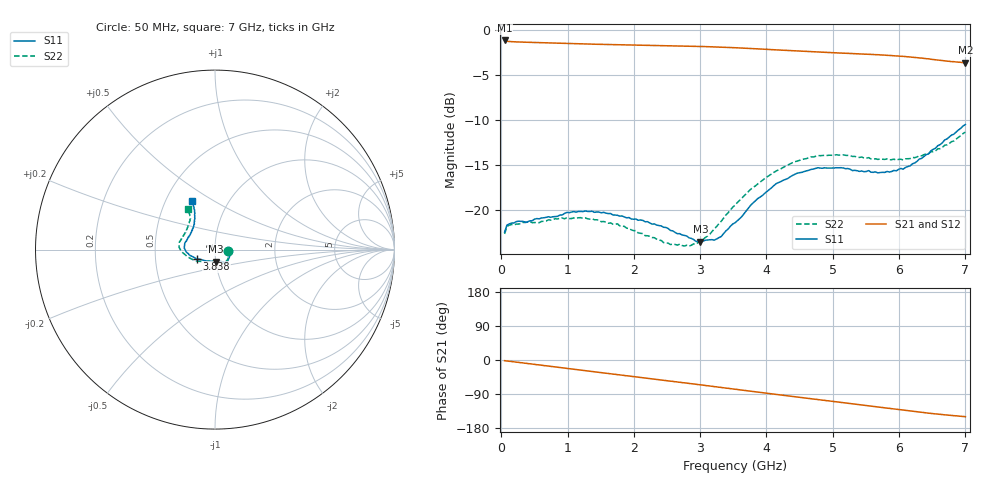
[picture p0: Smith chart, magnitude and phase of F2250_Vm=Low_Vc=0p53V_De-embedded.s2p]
! Integrated Device Technology
! Corporate Headquarters
! 6024 Silver Creek Valley Road
! San Jose, CA 95138  USA
! Phone:  1-408-284-8200
! Toll Free:  1-800-223-1366
! Webpage:  http://www.idt.com/
! Timing and RF Division
! 515 Groton Road, Suite 102
! Westford, MA 01886-6024
! Device:  F2250
! Description: Voltage Variable RF Attenuator
! Frequency:  50.0 -  6000.00 MHz
! Package:  3x3 mm Thin QFN Plastic Package: 16 pin
! Ports:  2 RF, 3 DC
!  Pin  1  = GND
!  Pin  2  = NC
!  Pin  3  = RF1  = Port 1
!  Pin  4  = NC
!  Pin  5  = GND
!  Pin  6  = GND
!  Pin  7  = GND
!  Pin  8  = GND
!  Pin  9  = NC
!  Pin 10  = RF2  = Port 2
!  Pin 11  = NC
!  Pin 12  = GND
!  Pin 13  = GND
!  Pin 14  = VCNTRL
!  Pin 15  = VDD
!  Pin 16  = VMODE
! Vcntrl:  0.530 Volts
! Vmode:  +0.000 Volts
! Vdd:  +3.30  Volts
! Current:  1.130 mA
! Data:  The device was measured on a the F2250 evaluation board which has
!  individual transmission lines to the RF pins.  Data was collected
!  using a calibrated network analyzer.  The evaluation board was
!  de-embedded using a TRL calibration technique.
!  The reference plane is the edge of the package pin.
! Misc:  SN 10
!  Action Tracker AT0258
! Date Measured:  2014-11-26
! Date:  2015-10-15  MJV
! Note:
!  Integrated Device Technology supplies this data as a sample of measured
!  data at the package pin for this product.  Your particular data for this
!  product may vary.
!  Data was taken at 25 degrees C.
!  Integrated Device Technology reserves the right to change this data at anytime.
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# GHz S dB R 50
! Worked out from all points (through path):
!   201 points, 50 MHz to 7 GHz, reference 50 ohm
!   highest |S21| = -1.12 dB at 50 MHz (marker M1); lowest = -3.6 dB at 7 GHz (marker M2)
!   group delay of S21, straight-line fit = 60.1 ps
!   lowest |S11| = -23.5 dB at 3.004 GHz (marker M3), VSWR 1.14, Z = 50 - j6.68 ohm
!   |S11| at or under -10 dB: start of sweep to end of sweep
!   |S22| runs from -24.0 to -11.3 dB; largest |S21 - S12| = 0.00041
!   S11 on the Smith chart (normalised r, x): 50 MHz: 1.16, -0.02; 3.838 GHz: 0.81, -0.08; 7 GHz: 0.68, +0.40
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0.05  -22.45 -7.3  -1.12 -1.8  -1.12 -1.8  -22.66 -8.3
0.08475  -21.68 -7.4  -1.20 -2.5  -1.20 -2.5  -21.83 -7.7
0.15425  -21.45 -9.4  -1.25 -4.0  -1.25 -4.0  -21.61 -9.5
0.71025  -20.75 -32.0  -1.39 -16.2  -1.39 -16.2  -21.09 -34.8
1.2315  -20.17 -48.1  -1.50 -27.4  -1.50 -27.4  -20.91 -54.9
1.75275  -20.58 -54.9  -1.60 -38.5  -1.60 -38.5  -21.54 -63.9
2.37825  -21.73 -57.0  -1.68 -51.8  -1.68 -51.8  -23.35 -70.6
2.552  -22.28 -60.4  -1.71 -55.6  -1.71 -55.6  -23.85 -76.4
2.83  -23.08 -72.2  -1.76 -61.7  -1.75 -61.7  -24.02 -92.9
3.00375  -23.52 -86.1  -1.79 -65.6  -1.79 -65.6  -23.40 -106.4
3.247  -23.23 -108.4  -1.84 -71.0  -1.84 -71.0  -21.84 -125.0
3.525  -21.42 -134.1  -1.93 -77.2  -1.93 -77.2  -19.46 -142.0
3.83775  -18.93 -152.9  -2.05 -84.1  -2.04 -84.1  -17.29 -156.4
4.1505  -17.05 -165.8  -2.17 -90.9  -2.17 -90.9  -15.64 -168.5
4.4285  -16.03 -174.4  -2.28 -97.0  -2.28 -97.0  -14.62 -176.1
4.7065  -15.43 178.5  -2.38 -103.0  -2.38 -103.0  -14.09 177.6
5.15825  -15.32 167.5  -2.54 -112.7  -2.54 -112.7  -13.85 168.0
5.85325  -15.76 143.8  -2.79 -127.6  -2.79 -127.7  -14.42 152.4
6.166  -15.09 132.1  -2.96 -134.4  -2.96 -134.5  -14.27 143.4
6.444  -13.74 122.9  -3.16 -140.2  -3.17 -140.3  -13.73 133.9
6.82625  -11.56 116.4  -3.48 -146.9  -3.48 -146.9  -12.32 125.8
7  -10.48 115.5  -3.60 -149.6  -3.61 -149.6  -11.32 124.3
